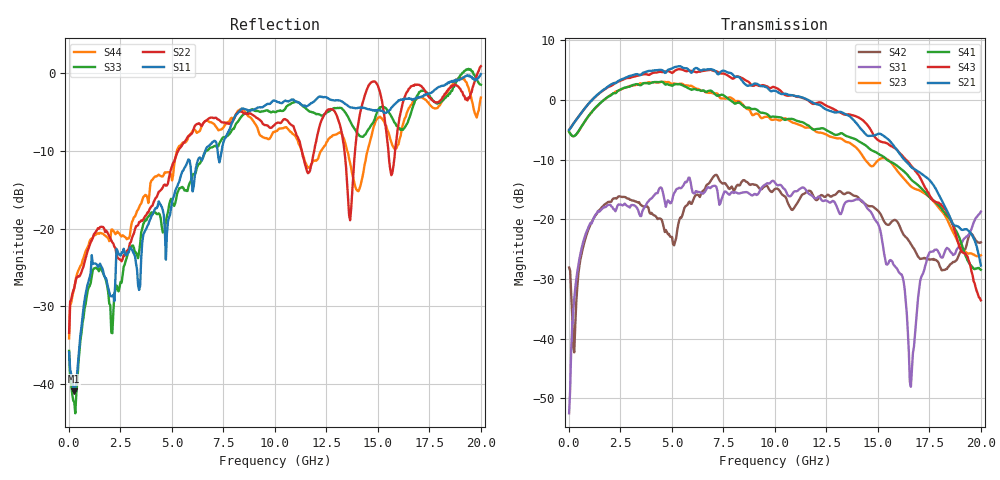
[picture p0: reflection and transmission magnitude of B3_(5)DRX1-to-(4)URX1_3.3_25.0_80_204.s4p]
!Agilent Technologies,N5225A,MY51451112,A.09.50.13
!Agilent N5225A: A.09.50.13
!Date: Sunday, March 12, 2017 05:22:52
!Correction: S11(Full 4 Port(1,2,3,4))
!S12(Full 4 Port(1,2,3,4))
!S13(Full 4 Port(1,2,3,4))
!S14(Full 4 Port(1,2,3,4))
!S21(Full 4 Port(1,2,3,4))
!S22(Full 4 Port(1,2,3,4))
!S23(Full 4 Port(1,2,3,4))
!S24(Full 4 Port(1,2,3,4))
!S31(Full 4 Port(1,2,3,4))
!S32(Full 4 Port(1,2,3,4))
!S33(Full 4 Port(1,2,3,4))
!S34(Full 4 Port(1,2,3,4))
!S41(Full 4 Port(1,2,3,4))
!S42(Full 4 Port(1,2,3,4))
!S43(Full 4 Port(1,2,3,4))
!S44(Full 4 Port(1,2,3,4))
!S4P File: Measurements: <S11,S12,S13,S14>,
!<S21,S22,S23,S24>,
!<S31,S32,S33,S34>,
!<S41,S42,S43,S44>:
# Hz S  dB  R 50
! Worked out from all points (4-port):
!   401 points, 10 MHz to 20 GHz, reference 50 ohm
!   strongest paths, dB at 10 MHz, 5.008 GHz, 10.01 GHz, 15 GHz, 20 GHz:
!     S21: -5.0, 5.3, 1.5, -5.7, -27.7
!     S43: -5.0, 4.5, 2.1, -6.7, -33.6
!     S41: -5.3, 2.4, -2.8, -9.0, -28.5
!     S23: -5.3, 2.7, -3.2, -10.1, -26.0
!     S31: -52.5, -16.9, -13.9, -20.7, -18.7
!     S42: -28.1, -23.0, -14.9, -18.5, -23.9
!   lowest |S11| = -40.9 dB at 259.9 MHz (marker M1), VSWR 1.02, Z = 50.3 - j0.863 ohm
!   |S11| at or under -10 dB: start of sweep to 6.627 GHz; 7.218 GHz to 7.417 GHz (198.7 MHz wide, 2.72 % of centre)
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1e7  -35.87 -37.1  -70.84 83.0  -54.08 10.6  -66.18 147.1
     -5.02 1.9  -33.39 39.2  -5.34 -179.5  -28.00 37.9
     -52.53 19.4  -75.24 123.7  -35.71 -45.5  -71.26 74.1
     -5.33 -179.5  -28.09 38.3  -5.00 2.0  -34.10 44.1
2.59875e8  -40.88 -71.8  -49.81 54.4  -33.09 94.9  -50.63 54.3
           -3.76 5.1  -27.63 -131.8  -6.03 179.5  -41.96 -162.8
           -33.23 95.4  -49.73 53.7  -42.27 -78.2  -50.49 55.6
           -6.03 178.7  -42.32 -170.3  -3.75 4.3  -27.67 -137.7
2.958525e9  -22.41 148.7  -43.11 -34.9  -17.65 52.1  -42.70 -60.4
            4.04 -94.2  -21.87 160.5  2.35 78.2  -16.76 38.8
            -18.03 54.4  -42.44 -31.2  -22.51 118.0  -41.27 -56.9
            2.24 68.6  -16.72 39.3  3.71 -101.9  -20.92 145.2
5.057475e9  -16.09 90.6  -41.14 10.5  -16.02 28.0  -39.26 -28.8
            5.42 169.5  -11.58 146.6  2.76 -26.0  -24.36 44.7
            -16.08 28.1  -37.72 -2.7  -16.91 102.1  -33.26 -41.0
            2.48 -41.1  -24.21 41.6  4.62 158.8  -13.17 126.5
8.2059e9  -5.16 36.3  -38.89 -114.3  -15.75 2.2  -36.76 -141.9
          3.91 13.2  -5.06 82.0  -0.15 -174.0  -13.88 47.1
          -15.64 1.4  -32.80 -112.9  -6.27 58.9  -32.00 -145.2
          -0.45 162.8  -14.20 51.4  3.94 0.4  -4.88 46.2
1.155422e10  -4.29 -6.1  -37.42 -117.9  -14.80 -22.3  -40.06 -137.0
             0.11 -131.7  -12.61 85.4  -4.61 43.4  -15.35 37.0
             -15.32 -23.5  -33.54 -122.9  -4.72 10.5  -34.08 -152.1
             -4.15 5.5  -15.37 42.4  0.06 -156.7  -11.89 25.4
2e10  -0.18 -114.1  -32.95 63.0  -18.73 121.2  -35.56 22.0
      -27.74 -162.2  0.84 17.1  -26.03 22.4  -23.89 102.0
      -18.71 121.2  -34.07 40.0  -1.53 -87.7  -35.28 -7.8
      -28.46 -25.8  -23.86 102.8  -33.59 167.9  -3.18 -136.7
